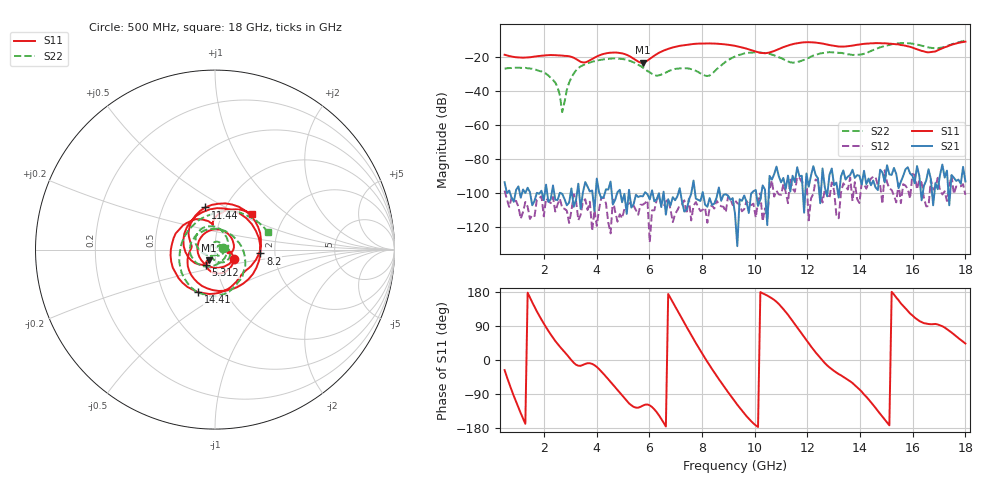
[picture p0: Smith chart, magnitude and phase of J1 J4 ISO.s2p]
!Agilent Technologies,N5230A,MY45001360,A.07.50.67
!Agilent N5230A: A.07.50.67
!Date: Tuesday, April 16, 2024 17:38:30
!Correction: S11(Full 2 Port(1,2))
!S21(Full 2 Port(1,2))
!S12(Full 2 Port(1,2))
!S22(Full 2 Port(1,2))
!S2P File: Measurements: S11, S21, S12, S22:
# Hz S  dB  R 50
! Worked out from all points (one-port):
!   201 points, 500 MHz to 18 GHz, reference 50 ohm
!   lowest |S11| = -23.3 dB at 5.75 GHz (marker M1), VSWR 1.15, Z = 46.3 - j5.51 ohm
!   |S11| at or under -10 dB: start of sweep to end of sweep
!   S11 on the Smith chart (normalised r, x): 500 MHz: 1.23, -0.13; 5.312 GHz: 0.89, -0.16; 8.2 GHz: 1.67, -0.08; 11.44 GHz: 0.81, +0.40; 14.41 GHz: 0.75, -0.38; 18 GHz: 1.38, +0.59
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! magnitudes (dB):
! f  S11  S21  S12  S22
! 500 MHz  -18.6  -93.5  -98.4  -26.8
! 2.075 GHz  -18.9  -94.9  -103.0  -29.7
! 2.513 GHz  -18.9  -104.0  -106.5  -37.7
! 2.6 GHz  -19.0  -99.7  -103.3  -42.6
! 2.688 GHz  -19.1  -100.3  -108.7  -52.3
! 2.95 GHz  -19.5  -105.5  -117.5  -34.9
! 3.475 GHz  -23.1  -99.4  -105.0  -24.8
! 4.438 GHz  -17.5  -97.8  -117.2  -21.0
! 5.312 GHz  -20.0  -108.4  -105.5  -22.5
! 5.75 GHz  -23.3  -101.8  -106.7  -26.1
! 6.362 GHz  -17.4  -100.0  -101.8  -30.7
! 7.412 GHz  -12.7  -109.7  -112.0  -26.5
! 8.2 GHz  -11.9  -107.9  -117.3  -31.1
! 9.25 GHz  -13.3  -112.1  -104.1  -19.6
! 10.39 GHz  -17.7  -97.8  -108.8  -17.6
! 11.44 GHz  -12.4  -89.7  -97.3  -23.2
! 12.22 GHz  -11.3  -84.1  -100.4  -19.1
! 13.28 GHz  -13.8  -90.1  -99.6  -17.5
! 14.41 GHz  -11.8  -95.3  -91.4  -16.4
! 15.11 GHz  -12.0  -88.9  -97.3  -12.8
! 16.6 GHz  -17.2  -85.9  -107.5  -14.3
! 18 GHz  -10.9  -93.1  -100.9  -10.2
